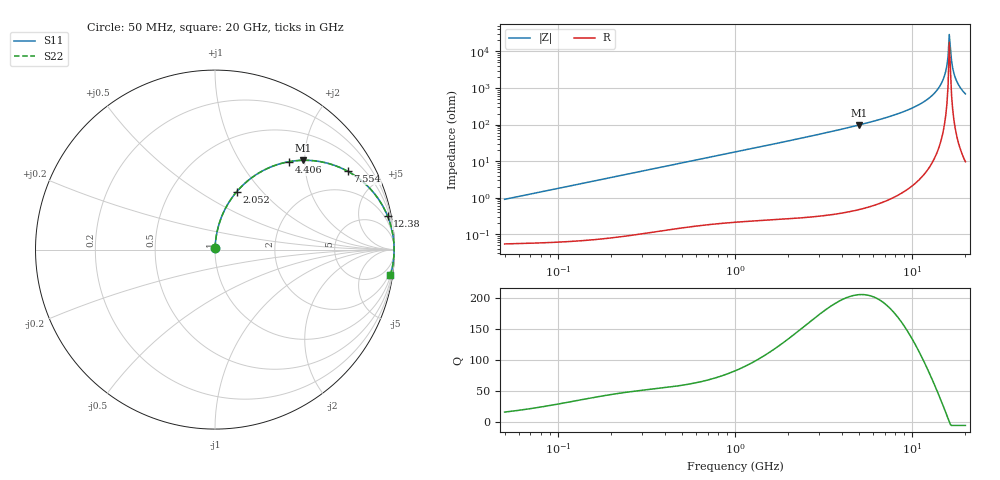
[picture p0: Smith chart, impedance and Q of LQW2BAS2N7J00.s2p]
!Murata Part Number: LQW2BAS2N7J00
!These Parameters are Measured in Series Mode Connection
!  o--[Z]--o
!Port1  Port2
!  o-------o
!Freq. Start=50[MHz] Stop=20[GHz], 401[Steps]
# Hz S RI R 50
!Freq.(Hz) S11(Real) S11(Imag) S21(Real) S21(Imag) S12(Real) S12(Imag) S22(Real) S22(Imag)
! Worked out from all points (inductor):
!   401 points, 50 MHz to 20 GHz, reference 50 ohm
!   read as one part in series: L = 2.87 nH near 51.52 MHz
!   highest Q = 206 at 5.041 GHz (marker M1), where L = 3.09 nH
!   self-resonance near 16.22 GHz
!   S11 on the Smith chart (normalised r, x): 50 MHz: 1.00, +0.02; 2.052 GHz: 1.01, +0.73; 4.406 GHz: 1.01, +1.67; 7.554 GHz: 1.02, +3.38; 12.38 GHz: 1, +10; 20 GHz: 1, -14
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5e7  0.000627 0.00902  0.9994 -0.00902  0.9994 -0.00902  0.000627 0.00902
1.364002e8  0.00127 0.0244  0.9987 -0.0244  0.9987 -0.0244  0.00127 0.0244
3.721004e8  0.00557 0.0658  0.9944 -0.0658  0.9944 -0.0658  0.00557 0.0658
1e9  0.0323 0.171  0.9677 -0.171  0.9677 -0.171  0.0323 0.171
2.05233e9  0.1203 0.3217  0.8797 -0.3217  0.8797 -0.3217  0.1203 0.3217
2.728004e9  0.1971 0.3948  0.8029 -0.3948  0.8029 -0.3948  0.1971 0.3948
4.405649e9  0.4112 0.4896  0.5888 -0.4896  0.5888 -0.4896  0.4112 0.4896
5.041459e9  0.4897 0.4975  0.5103 -0.4975  0.5103 -0.4975  0.4897 0.4975
7.442007e9  0.7308 0.4408  0.2692 -0.4408  0.2692 -0.4408  0.7308 0.4408
7.554318e9  0.7397 0.4361  0.2603 -0.4361  0.2603 -0.4361  0.7397 0.4361
1.004137e10  0.8883 0.3113  0.1117 -0.3113  0.1117 -0.3113  0.8883 0.3113
1.238412e10  0.9617 0.1859  0.0383 -0.1859  0.0383 -0.1859  0.9617 0.1859
1.375312e10  0.984 0.1164  0.016 -0.1164  0.016 -0.1164  0.984 0.1164
1.482269e10  0.9935 0.0651  0.00646 -0.0651  0.00646 -0.0651  0.9935 0.0651
1.550395e10  0.9967 0.034  0.00332 -0.034  0.00332 -0.034  0.9967 0.034
1.597544e10  0.9977 0.0131  0.00232 -0.0131  0.00232 -0.0131  0.9977 0.0131
1.621653e10  0.9979 0.00268  0.00214 -0.00268  0.00214 -0.00268  0.9979 0.00268
1.670968e10  0.9976 -0.0182  0.00245 0.0182  0.00245 0.0182  0.9976 -0.0182
1.721783e10  0.9964 -0.039  0.00363 0.039  0.00363 0.039  0.9964 -0.039
1.774144e10  0.9943 -0.0598  0.00568 0.0598  0.00568 0.0598  0.9943 -0.0598
1.88369e10  0.9876 -0.101  0.0124 0.101  0.0124 0.101  0.9876 -0.101
2e10  0.9775 -0.1415  0.0225 0.1415  0.0225 0.1415  0.9775 -0.1415
